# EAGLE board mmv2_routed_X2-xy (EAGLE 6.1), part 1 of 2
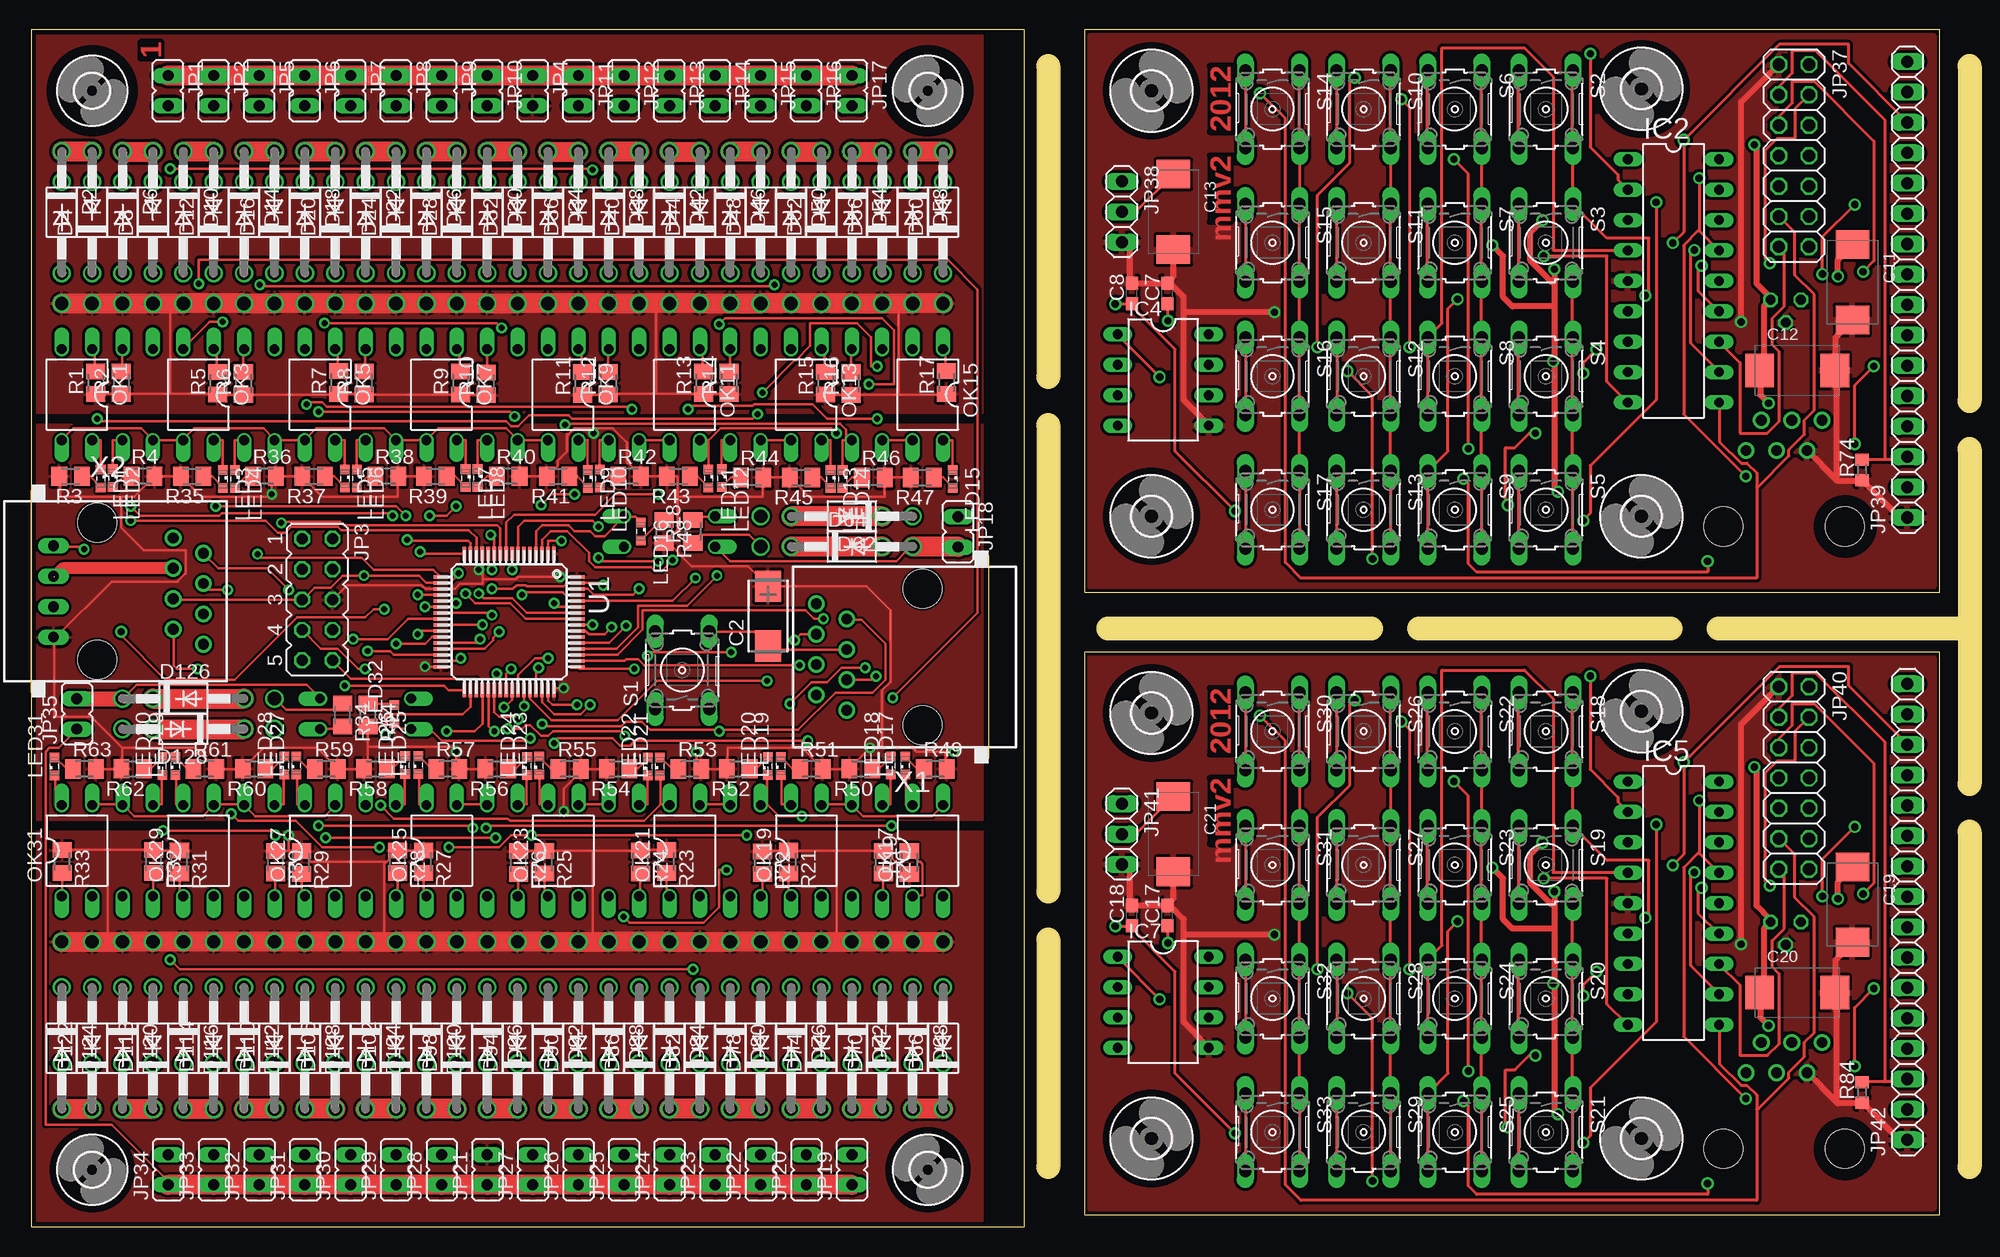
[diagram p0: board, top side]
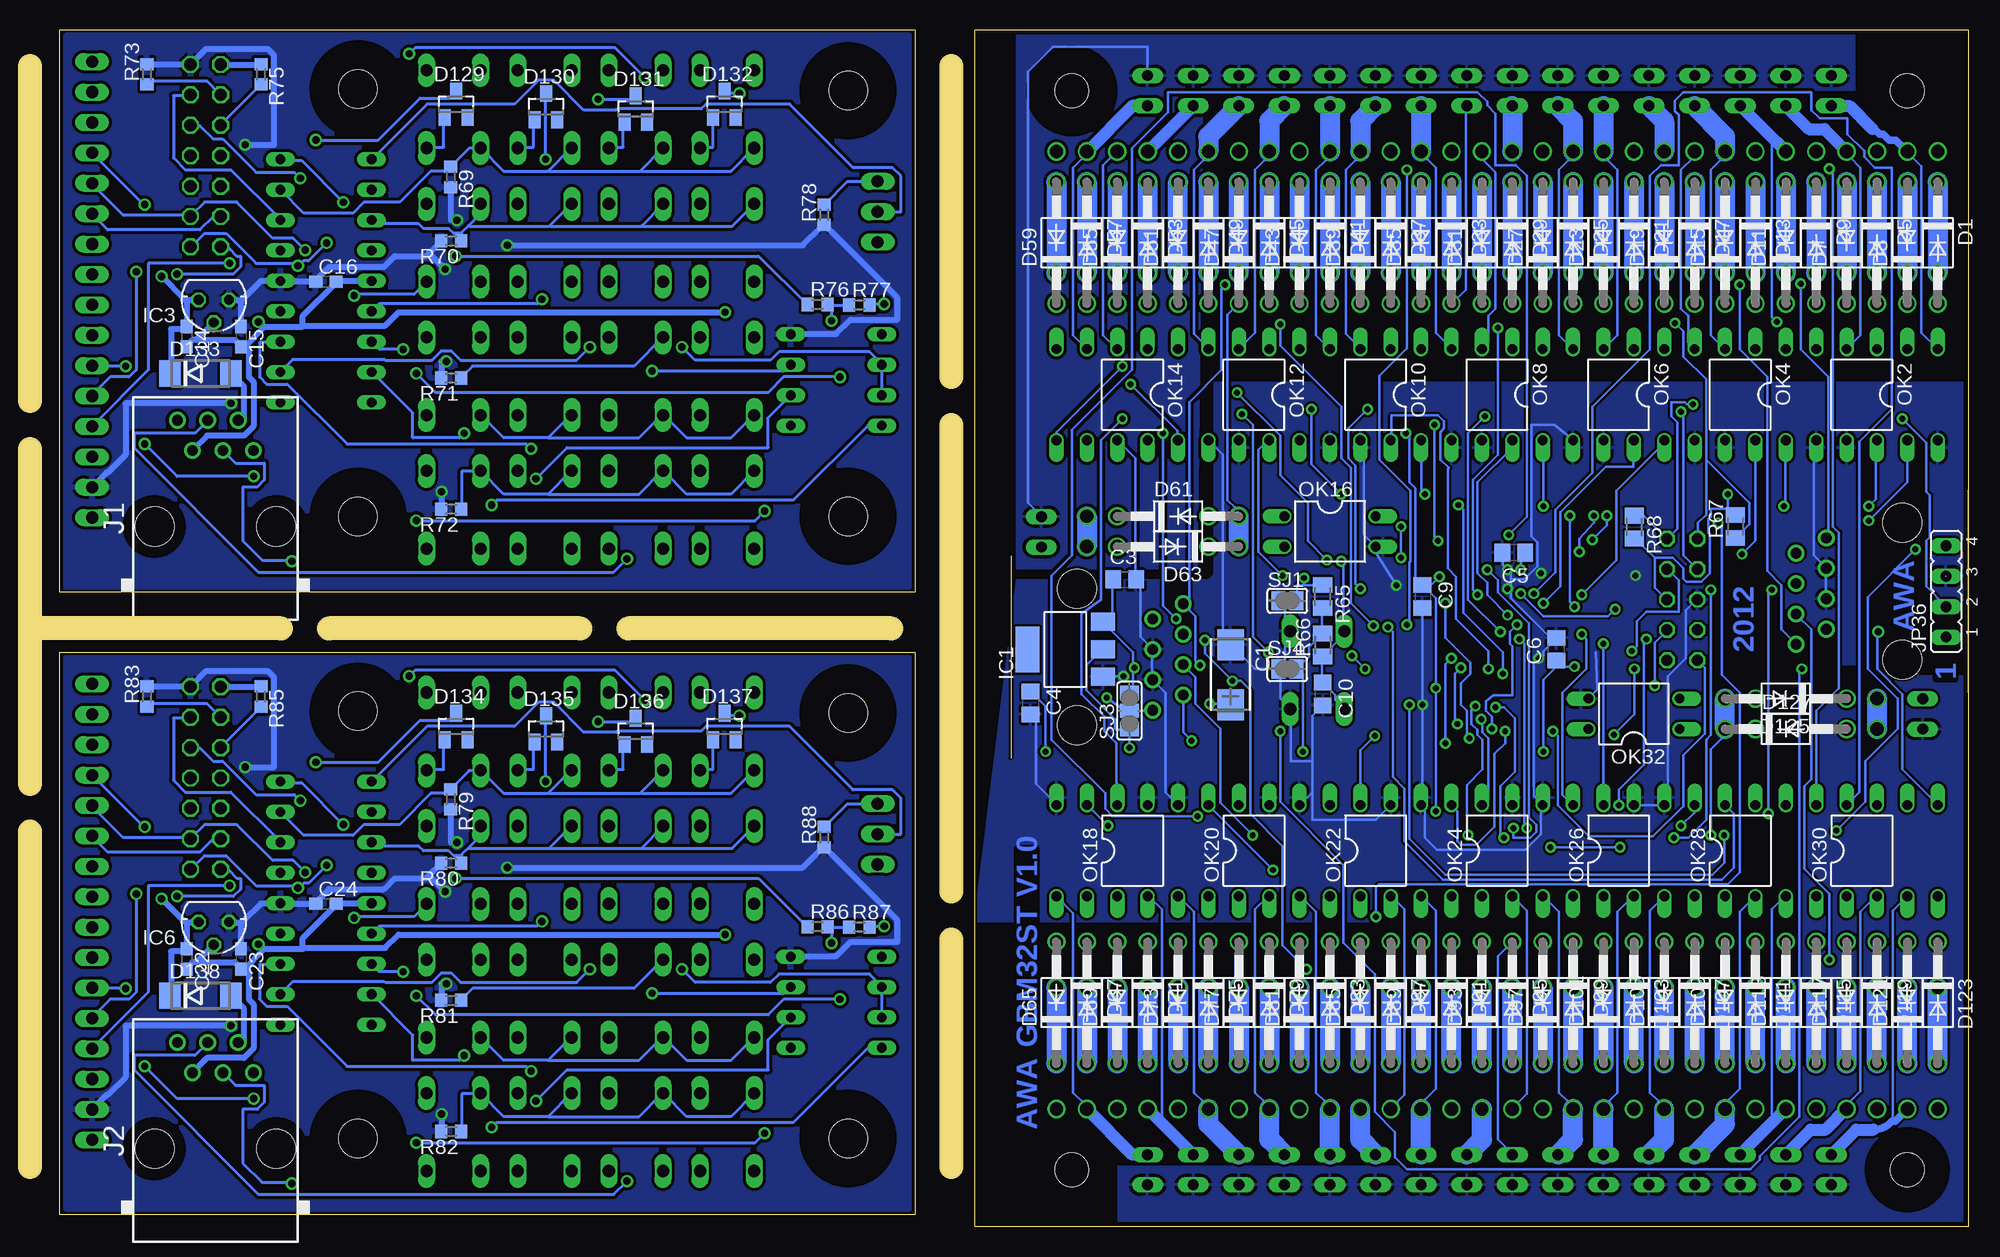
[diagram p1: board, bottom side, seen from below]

Size 162.02 x 100 mm. Coordinates in mm from the lower left corner, seen from the top.
Outline: 90.02,50 112.02,50
Outline: 116.02,50 137.02,50
Outline: 141.02,50 162.02,50
Outline: 162.02,97 162.02,69
Outline: 162.02,65 162.02,37
Outline: 162.02,33 162.02,5
Outline: 85.02,97 85.02,71
Outline: 85.02,67 85.02,28
Outline: 85.02,24 85.02,5
Outline: 0.01,100 0.01,0 83.01,0 83.01,100 0.01,100
Outline: 159.52,100 88.02,100 88.02,53 159.52,53 159.52,100
Outline: 159.52,48 88.02,48 88.02,1 159.52,1 159.52,48
Copper layers (1*16): Top 0.035mm / dielectric 1.5mm / Bottom 0.035mm
Design rules: minimum track width 0.2mm, minimum drill 0.5mm, track to track 0.2mm, track to pad 0.2mm, pad to pad 0.15mm, via to via 0.2mm, smd to smd 0mil, copper to edge 0.2mm, drill to drill 0.2mm, minimum pad ring 0.2mm, minimum via ring 0.2mm, stop-mask expansion 0.1mm, vias tented up to drill 0mil, thermal gap 10mil
Net classes: 1 Power: width 0.508 mm, clearance 0.254 mm

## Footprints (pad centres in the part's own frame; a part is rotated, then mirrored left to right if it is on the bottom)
CT6032 = smd 2.6 x 2.2: + 2.5,0; - -2.5,0
C0805 = smd 1.3 x 1.5: 1 -0.95,0; 2 0.95,0
C0603 = smd 1.1 x 1: 1 -0.85,0; 2 0.85,0
SMC_E = smd 2.4 x 2.8: + -3.15,0; - 3.15,0
DO41-10 = drill 1.118: A 5.08,0; C -5.08,0
SOT23 = smd 1 x 1.4: 1 -0.95,-1.1; 2 0.95,-1.1; 3 0,1.1
DO214AA = smd 1.8 x 2.2: A 2.55,0; C -2.55,0
2,8 = hole 2.8: 0,0
3,2 = hole 3.2: 0,0
SOT223 = smd 1.499 x 2.007: 1 -2.261,-3.15; 2 0.025,-3.15; 3 2.311,-3.15 | smd 3.81 x 2.007: 4 0,3.15
DIL18 = drill 0.813 long: 1 -10.16,-3.81; 2 -7.62,-3.81; 3 -5.08,-3.81; 4 -2.54,-3.81; 5 0,-3.81; 6 2.54,-3.81; 7 5.08,-3.81; 8 7.62,-3.81; 9 10.16,-3.81; 10 10.16,3.81; 11 7.62,3.81; 12 5.08,3.81; 13 2.54,3.81; 14 0,3.81; 15 -2.54,3.81; 16 -5.08,3.81; 17 -7.62,3.81; 18 -10.16,3.81
78LXX = drill 0.813 octagon: GND 0,1.905; IN 1.27,0; OUT -1.27,0
DIL08 = drill 0.813 long: 1 -3.81,-3.81; 2 -1.27,-3.81; 3 1.27,-3.81; 4 3.81,-3.81; 5 3.81,3.81; 6 1.27,3.81; 7 -1.27,3.81; 8 -3.81,3.81
RJ11-NO_SHIELD = drill 0.9 pad 1.4: 1 -3.175,8.89; 2 -1.905,6.35; 3 -0.635,8.89; 4 0.635,6.35; 5 1.905,8.89; 6 3.175,6.35 | hole 3.251: -5.08,0; 5.08,0
JP1 = drill 0.914 long: 1 0,-1.27; 2 0,1.27
JP5Q = drill 0.914 octagon: 1 -5.08,-1.27; 2 -5.08,1.27; 3 -2.54,-1.27; 4 -2.54,1.27; 5 0,-1.27; 6 0,1.27; 7 2.54,-1.27; 8 2.54,1.27; 9 5.08,-1.27; 10 5.08,1.27
JP4 = drill 0.914 long: 1 -3.81,0; 2 -1.27,0; 3 1.27,0; 4 3.81,0
2X07 = drill 1.016 octagon: 1 -7.62,-1.27; 2 -7.62,1.27; 3 -5.08,-1.27; 4 -5.08,1.27; 5 -2.54,-1.27; 6 -2.54,1.27; 7 0,-1.27; 8 0,1.27; 9 2.54,-1.27; 10 2.54,1.27; 11 5.08,-1.27; 12 5.08,1.27; 13 7.62,-1.27; 14 7.62,1.27
1X03 = drill 1.016 long: 1 -2.54,0; 2 0,0; 3 2.54,0
1X16 = drill 1.016 long: 1 -19.05,0; 2 -16.51,0; 3 -13.97,0; 4 -11.43,0; 5 -8.89,0; 6 -6.35,0; 7 -3.81,0; 8 -1.27,0; 9 1.27,0; 10 3.81,0; 11 6.35,0; 12 8.89,0; 13 11.43,0; 14 13.97,0; 15 16.51,0; 16 19.05,0
SML0603 = smd 0.8 x 0.8: A 0.75,0; C -0.75,0
DIL04 = drill 0.813 offset: 1 -1.27,-3.81; 2 1.27,-3.81; 3 1.27,3.81; 4 -1.27,3.81
M0805 = smd 1.3 x 1.6: 1 -0.95,0; 2 0.95,0
R0603 = smd 1 x 1.1: 1 -0.85,0; 2 0.85,0
B3F-10XX = drill 1.016 long: 1 -3.251,2.261; 2 3.251,2.261; 3 -3.251,-2.261; 4 3.251,-2.261
SJ = smd 1.168 x 1.6: 1 -0.762,0; 2 0.762,0
SJ_2 = smd 1.168 x 1.6: 1 -1.524,0; 2 0,0; 3 1.524,0
TQFP64 = smd 1.2 x 0.3: 1 -5.7,3.75; 2 -5.7,3.25; 3 -5.7,2.75; 4 -5.7,2.25; 5 -5.7,1.75; 6 -5.7,1.25; 7 -5.7,0.75; 8 -5.7,0.25; 9 -5.7,-0.25; 10 -5.7,-0.75; 11 -5.7,-1.25; 12 -5.7,-1.75; 13 -5.7,-2.25; 14 -5.7,-2.75; 15 -5.7,-3.25; 16 -5.7,-3.75; 33 5.7,-3.75; 34 5.7,-3.25; 35 5.7,-2.75; 36 5.7,-2.25; 37 5.7,-1.75; 38 5.7,-1.25; 39 5.7,-0.75; 40 5.7,-0.25; 41 5.7,0.25; 42 5.7,0.75; 43 5.7,1.25; 44 5.7,1.75; 45 5.7,2.25; 46 5.7,2.75; 47 5.7,3.25; 48 5.7,3.75 | smd 0.3 x 1.2: 17 -3.75,-5.7; 18 -3.25,-5.7; 19 -2.75,-5.7; 20 -2.25,-5.7; 21 -1.75,-5.7; 22 -1.25,-5.7; 23 -0.75,-5.7; 24 -0.25,-5.7; 25 0.25,-5.7; 26 0.75,-5.7; 27 1.25,-5.7; 28 1.75,-5.7; 29 2.25,-5.7; 30 2.75,-5.7; 31 3.25,-5.7; 32 3.75,-5.7; 49 3.75,5.7; 50 3.25,5.7; 51 2.75,5.7; 52 2.25,5.7; 53 1.75,5.7; 54 1.25,5.7; 55 0.75,5.7; 56 0.25,5.7; 57 -0.25,5.7; 58 -0.75,5.7; 59 -1.25,5.7; 60 -1.75,5.7; 61 -2.25,5.7; 62 -2.75,5.7; 63 -3.25,5.7; 64 -3.75,5.7
RJ45-NO-SHIELD = drill 0.9 pad 1.4: 1 -4.445,6.35; 2 -3.175,8.89; 3 -1.905,6.35; 4 -0.635,8.89; 5 0.635,6.35; 6 1.905,8.89; 7 3.175,6.35; 8 4.445,8.89 | hole 3.251: -5.715,0; 5.715,0

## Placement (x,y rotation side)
C1  [CT6032]  61.66,46.12 270 bottom
C2  [CT6032]  61.58,51.02 90 top
C3  [C0805]  70.5,54.08 0 bottom
C4  [C0805]  78.37,43.75 270 bottom
C5  [C0805]  37.99,56.32 180 bottom
C6  [C0805]  34.42,48.24 90 bottom
C7  100nF  [C0603]  94.96,77.98 90 top
C8  100nF  [C0603]  92,77.98 90 top
C9  [C0805]  45.61,52.65 270 bottom
C10  [C0805]  53.96,44.5 270 bottom
C11  100µF  [SMC_E]  152.23,78.91 270 top
C12  100µF  [SMC_E]  147.61,71.55 0 top
C13  10µF  [SMC_E]  95.47,84.8 270 top
C14  100nF  [C0603]  148.92,74.37 270 bottom
C15  100nF  [C0603]  144.38,74.37 270 bottom
C16  100nF  [C0603]  137.27,78.97 0 bottom
C17  100nF  [C0603]  94.96,25.98 90 top
C18  100nF  [C0603]  92,25.98 90 top
C19  100µF  [SMC_E]  152.23,26.91 270 top
C20  100µF  [SMC_E]  147.61,19.55 0 top
C21  10µF  [SMC_E]  95.47,32.8 270 top
C22  100nF  [C0603]  148.92,22.37 270 bottom
C23  100nF  [C0603]  144.38,22.37 270 bottom
C24  100nF  [C0603]  137.27,26.97 0 bottom
D1  1N4004  [DO41-10]  2.55,82.22 270 bottom
D2  1N4004  [DO41-10]  2.55,84.76 270 top
D3  1N4004  [DO41-10]  5.09,82.22 90 bottom
D4  1N4004  [DO41-10]  5.09,84.76 90 top
D5  1N4004  [DO41-10]  7.63,82.22 270 bottom
D6  1N4004  [DO41-10]  7.63,84.76 270 top
D7  1N4004  [DO41-10]  10.17,82.22 90 bottom
D8  1N4004  [DO41-10]  10.17,84.76 90 top
D9  1N4004  [DO41-10]  12.71,82.22 270 bottom
D10  1N4004  [DO41-10]  12.71,84.76 270 top
D11  1N4004  [DO41-10]  15.25,82.22 90 bottom
D12  1N4004  [DO41-10]  15.25,84.76 90 top
D13  1N4004  [DO41-10]  17.79,82.22 270 bottom
D14  1N4004  [DO41-10]  17.79,84.76 270 top
D15  1N4004  [DO41-10]  20.33,82.22 90 bottom
D16  1N4004  [DO41-10]  20.33,84.76 90 top
D17  1N4004  [DO41-10]  22.87,82.22 270 bottom
D18  1N4004  [DO41-10]  22.87,84.76 270 top
D19  1N4004  [DO41-10]  25.41,82.22 90 bottom
D20  1N4004  [DO41-10]  25.41,84.76 90 top
D21  1N4004  [DO41-10]  27.95,82.22 270 bottom
D22  1N4004  [DO41-10]  27.95,84.76 270 top
D23  1N4004  [DO41-10]  30.49,82.22 90 bottom
D24  1N4004  [DO41-10]  30.49,84.76 90 top
D25  1N4004  [DO41-10]  33.03,82.22 270 bottom
D26  1N4004  [DO41-10]  33.03,84.76 270 top
D27  1N4004  [DO41-10]  35.57,82.22 90 bottom
D28  1N4004  [DO41-10]  35.57,84.76 90 top
D29  1N4004  [DO41-10]  38.11,82.22 270 bottom
D30  1N4004  [DO41-10]  38.11,84.76 270 top
D31  1N4004  [DO41-10]  40.65,82.22 90 bottom
D32  1N4004  [DO41-10]  40.65,84.76 90 top
D33  1N4004  [DO41-10]  43.19,82.22 270 bottom
D34  1N4004  [DO41-10]  43.19,84.76 270 top
D35  1N4004  [DO41-10]  45.73,82.22 90 bottom
D36  1N4004  [DO41-10]  45.73,84.76 90 top
D37  1N4004  [DO41-10]  48.27,82.22 270 bottom
D38  1N4004  [DO41-10]  48.27,84.76 270 top
D39  1N4004  [DO41-10]  50.81,82.22 90 bottom
D40  1N4004  [DO41-10]  50.81,84.76 90 top
D41  1N4004  [DO41-10]  53.35,82.22 270 bottom
D42  1N4004  [DO41-10]  53.35,84.76 270 top
D43  1N4004  [DO41-10]  55.89,82.22 90 bottom
D44  1N4004  [DO41-10]  55.89,84.76 90 top
D45  1N4004  [DO41-10]  58.43,82.22 270 bottom
D46  1N4004  [DO41-10]  58.43,84.76 270 top
D47  1N4004  [DO41-10]  60.97,82.22 90 bottom
D48  1N4004  [DO41-10]  60.97,84.76 90 top
D49  1N4004  [DO41-10]  63.51,82.22 270 bottom
D50  1N4004  [DO41-10]  63.51,84.76 270 top
D51  1N4004  [DO41-10]  66.05,82.22 90 bottom
D52  1N4004  [DO41-10]  66.05,84.76 90 top
D53  1N4004  [DO41-10]  68.59,82.22 270 bottom
D54  1N4004  [DO41-10]  68.59,84.76 270 top
D55  1N4004  [DO41-10]  71.13,82.22 90 bottom
D56  1N4004  [DO41-10]  71.13,84.76 90 top
D57  1N4004  [DO41-10]  73.67,82.22 270 bottom
D58  1N4004  [DO41-10]  73.67,84.76 270 top
D59  1N4004  [DO41-10]  76.21,82.22 90 bottom
D60  1N4004  [DO41-10]  76.21,84.76 90 top
D61  1N4004  [DO41-10]  66.05,59.36 0 bottom
D62  1N4004  [DO41-10]  68.59,59.36 180 top
D63  1N4004  [DO41-10]  66.05,56.82 180 bottom
D64  1N4004  [DO41-10]  68.59,56.82 0 top
D65  1N4004  [DO41-10]  76.21,18.72 90 bottom
D66  1N4004  [DO41-10]  76.21,14.91 90 top
D67  1N4004  [DO41-10]  73.67,18.72 270 bottom
D68  1N4004  [DO41-10]  73.67,14.91 270 top
D69  1N4004  [DO41-10]  71.13,18.72 90 bottom
D70  1N4004  [DO41-10]  71.13,14.91 90 top
D71  1N4004  [DO41-10]  68.59,18.72 270 bottom
D72  1N4004  [DO41-10]  68.59,14.91 270 top
D73  1N4004  [DO41-10]  66.05,18.72 90 bottom
D74  1N4004  [DO41-10]  66.05,14.91 90 top
D75  1N4004  [DO41-10]  63.51,18.72 270 bottom
D76  1N4004  [DO41-10]  63.51,14.91 270 top
D77  1N4004  [DO41-10]  60.97,18.72 90 bottom
D78  1N4004  [DO41-10]  60.97,14.91 90 top
D79  1N4004  [DO41-10]  58.43,18.72 270 bottom
D80  1N4004  [DO41-10]  58.43,14.91 270 top
D81  1N4004  [DO41-10]  55.89,18.72 90 bottom
D82  1N4004  [DO41-10]  55.89,14.91 90 top
D83  1N4004  [DO41-10]  53.35,18.72 270 bottom
D84  1N4004  [DO41-10]  53.35,14.91 270 top
D85  1N4004  [DO41-10]  50.81,18.72 90 bottom
D86  1N4004  [DO41-10]  50.81,14.91 90 top
D87  1N4004  [DO41-10]  48.27,18.72 270 bottom
D88  1N4004  [DO41-10]  48.27,14.91 270 top
D89  1N4004  [DO41-10]  45.73,18.72 90 bottom
D90  1N4004  [DO41-10]  45.73,14.91 90 top
D91  1N4004  [DO41-10]  43.19,18.72 270 bottom
D92  1N4004  [DO41-10]  43.19,14.91 270 top
D93  1N4004  [DO41-10]  40.65,18.72 90 bottom
D94  1N4004  [DO41-10]  40.65,14.91 90 top
D95  1N4004  [DO41-10]  38.11,18.72 270 bottom
D96  1N4004  [DO41-10]  38.11,14.91 270 top
D97  1N4004  [DO41-10]  35.57,18.72 90 bottom
D98  1N4004  [DO41-10]  35.57,14.91 90 top
D99  1N4004  [DO41-10]  33.03,18.72 270 bottom
D100  1N4004  [DO41-10]  33.03,14.91 270 top
D101  1N4004  [DO41-10]  30.49,18.72 90 bottom
D102  1N4004  [DO41-10]  30.49,14.91 90 top
D103  1N4004  [DO41-10]  27.95,18.72 270 bottom
D104  1N4004  [DO41-10]  27.95,14.91 270 top
D105  1N4004  [DO41-10]  25.41,18.72 90 bottom
D106  1N4004  [DO41-10]  25.41,14.91 90 top
D107  1N4004  [DO41-10]  22.87,18.72 270 bottom
D108  1N4004  [DO41-10]  22.87,14.91 270 top
D109  1N4004  [DO41-10]  20.33,18.72 90 bottom
D110  1N4004  [DO41-10]  20.33,14.91 90 top
D111  1N4004  [DO41-10]  17.79,18.72 270 bottom
D112  1N4004  [DO41-10]  17.79,14.91 270 top
D113  1N4004  [DO41-10]  15.25,18.72 90 bottom
D114  1N4004  [DO41-10]  15.25,14.91 90 top
D115  1N4004  [DO41-10]  12.71,18.72 270 bottom
D116  1N4004  [DO41-10]  12.71,14.91 270 top
D117  1N4004  [DO41-10]  10.17,18.72 90 bottom
D118  1N4004  [DO41-10]  10.17,14.91 90 top
D119  1N4004  [DO41-10]  7.63,18.72 270 bottom
D120  1N4004  [DO41-10]  7.63,14.91 270 top
D121  1N4004  [DO41-10]  5.09,18.72 90 bottom
D122  1N4004  [DO41-10]  5.09,14.91 90 top
D123  1N4004  [DO41-10]  2.55,18.72 270 bottom
D124  1N4004  [DO41-10]  2.55,14.91 270 top
D125  1N4004  [DO41-10]  15.25,44.12 180 bottom
D126  1N4004  [DO41-10]  12.71,44.12 0 top
D127  1N4004  [DO41-10]  15.25,41.58 0 bottom
D128  1N4004  [DO41-10]  12.71,41.58 180 top
D129  BAV199  [SOT23]  126.4,93.79 0 bottom
D130  BAV199  [SOT23]  118.89,93.59 0 bottom
D131  BAV199  [SOT23]  111.38,93.39 0 bottom
D132  BAV199  [SOT23]  103.97,93.79 0 bottom
D133  [DO214AA]  147.76,71.29 0 bottom
D134  BAV199  [SOT23]  126.4,41.79 0 bottom
D135  BAV199  [SOT23]  118.89,41.59 0 bottom
D136  BAV199  [SOT23]  111.38,41.39 0 bottom
D137  BAV199  [SOT23]  103.97,41.79 0 bottom
D138  [DO214AA]  147.76,19.29 0 bottom
H1  MOUNT-HOLE2.8  [2,8]  5.09,94.92 270 top
H2  MOUNT-HOLE2.8  [2,8]  74.94,94.92 270 top
H3  MOUNT-HOLE2.8  [2,8]  5.09,4.75 270 top
H4  MOUNT-HOLE2.8  [2,8]  74.94,4.75 270 top
H5  MOUNT-HOLE3.2  [3,2]  134.59,59.36 180 top
H6  MOUNT-HOLE3.2  [3,2]  93.63,59.36 180 top
H7  MOUNT-HOLE3.2  [3,2]  134.59,95.07 180 top
H8  MOUNT-HOLE3.2  [3,2]  93.63,94.92 180 top
H9  MOUNT-HOLE3.2  [3,2]  134.59,7.36 180 top
H10  MOUNT-HOLE3.2  [3,2]  93.63,7.36 180 top
H11  MOUNT-HOLE3.2  [3,2]  134.59,43.07 180 top
H12  MOUNT-HOLE3.2  [3,2]  93.63,42.92 180 top
IC1  REG1117  [SOT223]  75.48,48.22 90 bottom
IC2  PIC16F628P  [DIL18]  137.27,79.03 270 top
IC3  [78LXX]  146.65,77.45 180 bottom
IC4  MAX481CPA  [DIL08]  94.62,70.75 270 top
IC5  PIC16F628P  [DIL18]  137.27,27.03 270 top
IC6  [78LXX]  146.65,25.45 180 bottom
IC7  MAX481CPA  [DIL08]  94.62,18.75 270 top
J1  RJ11-6L-B  [RJ11-NO_SHIELD]  146.52,58.5 0 bottom
J2  RJ11-6L-B  [RJ11-NO_SHIELD]  146.52,6.5 0 bottom
JP1  [JP1]  11.44,94.92 180 top
JP2  [JP1]  15.25,94.92 180 top
JP3  [JP5Q]  23.91,52.4 270 top
JP4  [JP1]  41.92,94.92 180 top
JP5  [JP1]  19.06,94.92 180 top
JP6  [JP1]  22.87,94.92 180 top
JP7  [JP1]  26.68,94.92 180 top
JP8  [JP1]  30.49,94.92 180 top
JP9  [JP1]  34.3,94.92 180 top
JP10  [JP1]  38.11,94.92 180 top
JP11  [JP1]  45.73,94.92 180 top
JP12  [JP1]  49.54,94.92 180 top
JP13  [JP1]  53.35,94.92 180 top
JP14  [JP1]  57.16,94.92 180 top
JP15  [JP1]  60.97,94.92 180 top
JP16  [JP1]  64.78,94.92 180 top
JP17  [JP1]  68.59,94.92 180 top
JP18  [JP1]  77.48,58.06 180 top
JP19  [JP1]  68.59,4.75 0 top
JP20  [JP1]  64.78,4.75 0 top
JP21  [JP1]  38.11,4.75 0 top
JP22  [JP1]  60.97,4.75 0 top
JP23  [JP1]  57.16,4.75 0 top
JP24  [JP1]  53.35,4.75 0 top
JP25  [JP1]  49.54,4.75 0 top
JP26  [JP1]  45.73,4.75 0 top
JP27  [JP1]  41.92,4.75 0 top
JP28  [JP1]  34.3,4.75 0 top
JP29  [JP1]  30.49,4.75 0 top
JP30  [JP1]  26.68,4.75 0 top
JP31  [JP1]  22.87,4.75 0 top
JP32  [JP1]  19.06,4.75 0 top
JP33  [JP1]  15.25,4.75 0 top
JP34  [JP1]  11.44,4.75 0 top
JP35  [JP1]  3.82,42.85 0 top
JP36  [JP4]  1.86,53.08 90 bottom
JP37  [2X07]  147.33,89.49 270 top
JP38  [1X03]  91.16,84.8 270 top
JP39  [1X16]  156.82,78.3 90 top
JP40  [2X07]  147.33,37.49 270 top
JP41  [1X03]  91.16,32.8 270 top
JP42  [1X16]  156.82,26.3 90 top
LED1  [SML0603]  5.81,62.52 270 top
LED2  [SML0603]  6.81,62.54 270 top
LED3  [SML0603]  16.01,62.46 270 top
LED4  [SML0603]  17.01,62.48 270 top
LED5  [SML0603]  26.21,62.5 270 top
LED6  [SML0603]  27.21,62.52 270 top
LED7  [SML0603]  36.31,62.54 270 top
LED8  [SML0603]  37.31,62.56 270 top
LED9  [SML0603]  46.51,62.48 270 top
LED10  [SML0603]  47.51,62.5 270 top
LED11  [SML0603]  56.61,62.52 270 top
LED12  [SML0603]  57.71,62.54 270 top
LED13  [SML0603]  66.81,62.46 270 top
LED14  [SML0603]  67.81,62.48 270 top
LED15  [SML0603]  77.01,62.47 270 top
LED16  [SML0603]  50.96,58.09 270 top
LED17  [SML0603]  73.05,38.54 90 top
LED18  [SML0603]  71.85,38.52 90 top
LED19  [SML0603]  62.65,38.5 90 top
LED20  [SML0603]  61.55,38.48 90 top
LED21  [SML0603]  52.55,38.46 90 top
LED22  [SML0603]  51.55,38.44 90 top
LED23  [SML0603]  42.45,38.52 90 top
LED24  [SML0603]  41.45,38.5 90 top
LED25  [SML0603]  32.35,38.58 90 top
LED26  [SML0603]  31.25,38.56 90 top
LED27  [SML0603]  22.15,38.54 90 top
LED28  [SML0603]  21.15,38.52 90 top
LED29  [SML0603]  12.05,38.5 90 top
LED30  [SML0603]  10.95,38.48 90 top
LED31  [SML0603]  1.95,38.46 90 top
LED32  [SML0603]  30.37,42.85 90 top
OK1  PC817  [DIL04]  3.82,69.52 180 top
OK2  PC817  [DIL04]  8.9,69.52 180 bottom
OK3  PC817  [DIL04]  13.98,69.52 180 top
OK4  PC817  [DIL04]  19.06,69.52 180 bottom
OK5  PC817  [DIL04]  24.14,69.52 180 top
OK6  PC817  [DIL04]  29.22,69.52 180 bottom
OK7  PC817  [DIL04]  34.3,69.52 180 top
OK8  PC817  [DIL04]  39.38,69.52 180 bottom
OK9  PC817  [DIL04]  44.46,69.52 180 top
OK10  PC817  [DIL04]  49.54,69.52 180 bottom
OK11  PC817  [DIL04]  54.62,69.52 180 top
OK12  PC817  [DIL04]  59.7,69.52 180 bottom
OK13  PC817  [DIL04]  64.78,69.52 180 top
OK14  PC817  [DIL04]  69.86,69.52 180 bottom
OK15  PC817  [DIL04]  74.94,69.52 180 top
OK16  PC817  [DIL04]  53.35,58.09 270 bottom
OK17  PC817  [DIL04]  74.94,31.42 0 top
OK18  PC817  [DIL04]  69.86,31.42 0 bottom
OK19  PC817  [DIL04]  64.78,31.42 0 top
OK20  PC817  [DIL04]  59.7,31.42 0 bottom
OK21  PC817  [DIL04]  54.62,31.42 0 top
OK22  PC817  [DIL04]  49.54,31.42 0 bottom
OK23  PC817  [DIL04]  44.46,31.42 0 top
OK24  PC817  [DIL04]  39.38,31.42 0 bottom
OK25  PC817  [DIL04]  34.3,31.42 0 top
OK26  PC817  [DIL04]  29.22,31.42 0 bottom
OK27  PC817  [DIL04]  24.14,31.42 0 top
OK28  PC817  [DIL04]  19.06,31.42 0 bottom
OK29  PC817  [DIL04]  13.98,31.42 0 top
OK30  PC817  [DIL04]  8.9,31.42 0 bottom
OK31  PC817  [DIL04]  3.82,31.42 0 top
OK32  PC817  [DIL04]  27.95,42.85 90 bottom
R1  680R  [M0805]  5.39,70.51 90 top
R2  680R  [M0805]  7.53,70.51 90 top
R3  [M0805]  3.29,62.7 180 top
R4  [M0805]  9.35,62.7 0 top
R5  680R  [M0805]  15.59,70.47 90 top
R6  680R  [M0805]  17.73,70.45 90 top
R7  680R  [M0805]  25.69,70.53 90 top
R8  680R  [M0805]  27.83,70.49 90 top
R9  680R  [M0805]  35.89,70.49 90 top
R10  680R  [M0805]  38.03,70.43 90 top
R11  680R  [M0805]  46.09,70.45 90 top
R12  680R  [M0805]  48.23,70.47 90 top
R13  680R  [M0805]  56.19,70.51 90 top
R14  680R  [M0805]  58.33,70.51 90 top
R15  680R  [M0805]  66.39,70.47 90 top
R16  680R  [M0805]  68.53,70.45 90 top
R17  680R  [M0805]  76.49,70.53 90 top
R18  680R  [M0805]  55.3,58.09 90 top
R19  680R  [M0805]  73.39,30.43 90 top
R20  680R  [M0805]  71.23,30.45 270 top
R21  680R  [M0805]  63.29,30.47 270 top
R22  680R  [M0805]  61.13,30.41 270 top
R23  680R  [M0805]  53.09,30.51 270 top
R24  680R  [M0805]  50.93,30.47 270 top
R25  680R  [M0805]  42.89,30.45 270 top
R26  680R  [M0805]  40.73,30.43 270 top
R27  680R  [M0805]  32.79,30.49 270 top
R28  680R  [M0805]  30.63,30.49 270 top
R29  680R  [M0805]  22.59,30.43 270 top
R30  680R  [M0805]  20.43,30.45 270 top
R31  680R  [M0805]  12.39,30.47 270 top
R32  680R  [M0805]  10.23,30.51 270 top
R33  680R  [M0805]  2.59,30.51 270 top
R34  680R  [M0805]  26.02,42.75 270 top
R35  [M0805]  13.45,62.7 180 top
R36  [M0805]  19.49,62.7 0 top
R37  [M0805]  23.61,62.7 180 top
R38  [M0805]  29.73,62.7 0 top
R39  [M0805]  33.77,62.7 180 top
R40  [M0805]  39.87,62.7 0 top
R41  [M0805]  44.03,62.7 180 top
R42  [M0805]  50.01,62.7 0 top
R43  [M0805]  54.09,62.7 180 top
R44  [M0805]  60.25,62.6 0 top
R45  [M0805]  64.35,62.6 180 top
R46  [M0805]  70.39,62.6 0 top
R47  [M0805]  74.48,62.6 180 top
R48  [M0805]  52.91,58.09 270 top
R49  [M0805]  75.57,38.24 0 top
R50  [M0805]  69.33,38.26 180 top
R51  [M0805]  65.21,38.24 0 top
R52  [M0805]  59.09,38.26 180 top
R53  [M0805]  55.05,38.24 0 top
R54  [M0805]  49.05,38.26 180 top
R55  [M0805]  44.99,38.24 0 top
R56  [M0805]  38.91,38.26 180 top
R57  [M0805]  34.83,38.24 0 top
R58  [M0805]  28.77,38.26 180 top
R59  [M0805]  24.67,38.24 0 top
R60  [M0805]  18.63,38.26 180 top
R61  [M0805]  14.51,38.24 0 top
R62  [M0805]  8.49,38.26 180 top
R63  [M0805]  4.45,38.24 0 top
R64  [M0805]  28.15,42.75 270 top
R65  10k  [M0805]  53.96,52.65 270 bottom
R66  10k  [M0805]  53.96,48.6 90 bottom
R67  10k  [M0805]  19.46,58.5 90 bottom
R68  10k  [M0805]  27.91,58.45 270 bottom
R69  10k  [R0603]  126.85,87.71 270 bottom
R70  10k  [R0603]  126.81,82.37 180 bottom
R71  10k  [R0603]  126.81,70.91 180 bottom
R72  10k  [R0603]  126.81,59.95 180 bottom
R73  10k  [R0603]  152.24,96.3 90 bottom
R74  330R  [R0603]  153.03,63.22 90 top
R75  0R  [R0603]  142.7,96.3 270 bottom
R76  2k7  [R0603]  96.19,77.06 0 bottom
R77  2k7  [R0603]  92.69,77.02 0 bottom
R78  5k6  [R0603]  95.63,84.55 90 bottom
R79  10k  [R0603]  126.85,35.71 270 bottom
R80  10k  [R0603]  126.81,30.37 180 bottom
R81  10k  [R0603]  126.81,18.91 180 bottom
R82  10k  [R0603]  126.81,7.95 180 bottom
R83  10k  [R0603]  152.24,44.3 90 bottom
R84  330R  [R0603]  153.03,11.22 90 top
R85  0R  [R0603]  142.7,44.3 270 bottom
R86  2k7  [R0603]  96.19,25.06 0 bottom
R87  2k7  [R0603]  92.69,25.02 0 bottom
R88  5k6  [R0603]  95.63,32.55 90 bottom
S1  [B3F-10XX]  54.41,46.5 90 top
S2  [B3F-10XX]  126.61,93.38 270 top
S3  [B3F-10XX]  126.61,82.22 270 top
S4  [B3F-10XX]  126.61,71.06 270 top
S5  [B3F-10XX]  126.61,59.9 270 top
S6  [B3F-10XX]  118.99,93.38 270 top
S7  [B3F-10XX]  118.99,82.22 270 top
S8  [B3F-10XX]  118.99,71.06 270 top
S9  [B3F-10XX]  118.99,59.9 270 top
S10  [B3F-10XX]  111.37,93.38 270 top
S11  [B3F-10XX]  111.37,82.22 270 top
S12  [B3F-10XX]  111.37,71.06 270 top
S13  [B3F-10XX]  111.37,59.9 270 top
S14  [B3F-10XX]  103.75,93.38 270 top
S15  [B3F-10XX]  103.75,82.22 270 top
S16  [B3F-10XX]  103.75,71.06 270 top
S17  [B3F-10XX]  103.75,59.9 270 top
S18  [B3F-10XX]  126.61,41.38 270 top
S19  [B3F-10XX]  126.61,30.22 270 top
S20  [B3F-10XX]  126.61,19.06 270 top
S21  [B3F-10XX]  126.61,7.9 270 top
S22  [B3F-10XX]  118.99,41.38 270 top
S23  [B3F-10XX]  118.99,30.22 270 top
S24  [B3F-10XX]  118.99,19.06 270 top
S25  [B3F-10XX]  118.99,7.9 270 top
S26  [B3F-10XX]  111.37,41.38 270 top
S27  [B3F-10XX]  111.37,30.22 270 top
S28  [B3F-10XX]  111.37,19.06 270 top
S29  [B3F-10XX]  111.37,7.9 270 top
S30  [B3F-10XX]  103.75,41.38 270 top
S31  [B3F-10XX]  103.75,30.22 270 top
S32  [B3F-10XX]  103.75,19.06 270 top
S33  [B3F-10XX]  103.75,7.9 270 top
SJ1  [SJ]  56.91,52.3 0 bottom
SJ3  [SJ_2]  70.11,43.1 90 bottom
SJ4  [SJ]  56.91,46.6 0 bottom
U1  STM32F10XRXT6  [TQFP64]  39.94,50.53 270 top
X1  RJ45-6L-B  [RJ45-NO-SHIELD]  74.51,47.6 90 top
X2  RJ45-6L-B  [RJ45-NO-SHIELD]  5.51,53.1 270 top

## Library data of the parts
C1 C2 R1-R68 = resistor
C3-C24 R69-R88 = rcl
D1-D138 = diode
H1-H12 = holes
IC1 = burr-brown; MPN: REG1117; OC_FARNELL: 1097566; OC_NEWARK: 14P6981
IC2 IC5 = microchip; MF: MICROCHIP; MPN: PIC16F628-20/P; OC_FARNELL: 9760423; OC_NEWARK: 23C4982
IC3 IC6 = v-reg
IC4 IC7 = maxim; MPN: MAX481CPA+; OC_FARNELL: unknown; OC_NEWARK: 99K3445
J1 J2 = con-tycoelectronics_local; MF: TYCO ELECTRONICS; MPN: RJ11-6L-B; OC_FARNELL: unknown; OC_NEWARK: 52K3613
JP1-JP36 SJ1 SJ3 SJ4 = jumper
JP37-JP42 = pinhead
LED1-LED32 = led
OK1-OK32 = optocoupler; MPN: PC817X4J000F; OC_FARNELL: 9707727; OC_NEWARK: 97K7059
S1-S33 = switch-omron; MPN: B3F-1000; OC_FARNELL: 176432; OC_NEWARK: 36M3542
U1 = stm32
X1 X2 = con-tycoelectronics; MPN: RJ45-6L-B; OC_FARNELL: unknown; OC_NEWARK: 16R6090

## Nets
COL1: IC2.17 R69.1 S2.3 S2.4 S6.3 S6.4 S10.3 S10.4 S14.3 S14.4
COL2: IC2.3 R70.1 S3.3 S3.4 S7.3 S7.4 S11.3 S11.4 S15.3 S15.4
COL3: IC2.4 R71.1 S4.3 S4.4 S8.3 S8.4 S12.3 S12.4 S16.3 S16.4
COL4: IC2.6 R72.1 S5.3 S5.4 S9.3 S9.4 S13.3 S13.4 S17.3 S17.4
COL5: IC5.17 R79.1 S18.3 S18.4 S22.3 S22.4 S26.3 S26.4 S30.3 S30.4
COL6: IC5.3 R80.1 S19.3 S19.4 S23.3 S23.4 S27.3 S27.4 S31.3 S31.4
COL7: IC5.4 R81.1 S20.3 S20.4 S24.3 S24.4 S28.3 S28.4 S32.3 S32.4
COL8: IC5.6 R82.1 S21.3 S21.4 S25.3 S25.4 S29.3 S29.4 S33.3 S33.4
DB1: D137.3 IC5.10 JP40.11 JP42.11
DB2: D135.3 IC5.12 JP40.13 JP42.13
DB3: D136.3 IC5.11 JP40.12 JP42.12
DB4: D132.3 IC2.10 JP37.11 JP39.11
DB5: D131.3 IC2.11 JP37.12 JP39.12
DB6: D130.3 IC2.12 JP37.13 JP39.13
DB7: D129.3 IC2.13 JP37.14 JP39.14
DB8: D134.3 IC5.13 JP40.14 JP42.14
DIR: IC2.2 IC4.2 IC4.3
DIR1: IC5.2 IC7.2 IC7.3
E: IC2.15 JP37.6 JP39.6
E1: IC5.15 JP40.6 JP42.6
GBM0: LED1.C OK1.4 U1.14
GBM1: LED2.C OK2.4 U1.15
GBM2: LED3.C OK3.4 U1.16
GBM3: LED4.C OK4.4 U1.17
GBM4: LED5.C OK5.4 U1.20
GBM5: LED6.C OK6.4 U1.21
GBM6: LED7.C OK7.4 U1.22
GBM7: LED8.C OK8.4 U1.23
GBM8: LED9.C OK9.4 U1.39
GBM9: LED10.C OK10.4 U1.40
GBM10: LED11.C OK11.4 U1.51
GBM11: LED12.C OK12.4 U1.52
GBM12: LED13.C OK13.4 U1.53
GBM13: LED14.C OK14.4 U1.2
GBM14: LED15.C OK15.4 U1.3
GBM15: LED16.C OK16.4 U1.4
GBM16: LED17.C OK17.4 U1.8
GBM17: LED18.C OK18.4 U1.9
GBM18: LED19.C OK19.4 U1.10
GBM19: LED20.C OK20.4 U1.11
GBM20: LED21.C OK21.4 U1.24
GBM21: LED22.C OK22.4 U1.25
GBM22: LED23.C OK23.4 U1.37
GBM23: LED24.C OK24.4 U1.38
GBM24: LED25.C OK25.4 U1.26
GBM25: LED26.C OK26.4 U1.27
GBM26: LED27.C OK27.4 U1.28
GBM27: LED28.C OK28.4 U1.55
GBM28: LED29.C OK29.4 U1.56
GBM29: LED30.C OK30.4 U1.57
GBM30: LED31.C OK31.4 U1.58
GBM31: LED32.C OK32.4 U1.59
GLC1N: JP19.1 JP20.1 JP21.1 JP22.1 JP23.1 JP24.1 JP25.1 JP26.1 JP27.1 JP28.1 JP29.1 JP30.1 JP31.1 JP32.1 JP33.1 JP34.1 JP35.1
GLC1P: D65.A D67.C D69.A D71.C D73.A D75.C D77.A D79.C D81.A D83.C D85.A D87.C D89.A D91.C D93.A D95.C D97.A D99.C D101.A D103.C D105.A D107.C D109.A D111.C D113.A D115.C D117.A D119.C D121.A D123.C D125.A D127.C JP21.2 R19.1 R20.1 R21.1 R22.1 R23.1 R24.1 R25.1 R26.1 R27.1 R28.1 R29.1 R30.1 R31.1 R32.1 R33.1 R34.1
GLCN: JP1.1 JP2.1 JP4.1 JP5.1 JP6.1 JP7.1 JP8.1 JP9.1 JP10.1 JP11.1 JP12.1 JP13.1 JP14.1 JP15.1 JP16.1 JP17.1 JP18.1
GLCP: D1.A D3.C D5.A D7.C D9.A D11.C D13.A D15.C D17.A D19.C D21.A D23.C D25.A D27.C D29.A D31.C D33.A D35.C D37.A D39.C D41.A D43.C D45.A D47.C D49.A D51.C D53.A D55.C D57.A D59.C D61.A D63.C JP4.2 R1.1 R2.1 R5.1 R6.1 R7.1 R8.1 R9.1 R10.1 R11.1 R12.1 R13.1 R14.1 R15.1 R16.1 R17.1 R18.1
GND: C1.- C2.- C3.2 C4.2 C5.2 C6.2 C9.2 C10.2 IC1.1 JP3.5 JP36.3 OK1.3 OK2.3 OK3.3 OK4.3 OK5.3 OK6.3 OK7.3 OK8.3 OK9.3 OK10.3 OK11.3 OK12.3 OK13.3 OK14.3 OK15.3 OK16.3 OK17.3 OK18.3 OK19.3 OK20.3 OK21.3 OK22.3 OK23.3 OK24.3 OK25.3 OK26.3 OK27.3 OK28.3 OK29.3 OK30.3 OK31.3 OK32.3 S1.3 S1.4 SJ1.1 SJ4.1 U1.12 U1.18 U1.31 U1.47 U1.63 X1.3 X1.5 X2.3 X2.5
GND1 [Power]: C7.2 C8.2 C11.- C12.- C13.- C14.2 C15.2 C16.2 IC2.5 IC3.GND IC4.5 J1.2 JP37.1 JP38.3 JP39.1 R74.1 R75.1
GND2 [Power]: C17.2 C18.2 C19.- C20.- C21.- C22.2 C23.2 C24.2 IC5.5 IC6.GND IC7.5 J2.2 JP40.1 JP41.3 JP42.1 R84.1 R85.1
I2C_SCL: JP3.1 R67.1 U1.61
I2C_SDA: JP3.2 R68.1 U1.62
MES: C8.1 IC2.18 R77.2
MES1: C18.1 IC5.18 R87.2
N$1: R65.1 SJ1.2 U1.60
N$2: D3.A D4.C
N$3: D1.C D2.A
N$4: D2.C D4.A JP1.2 OK1.2
N$5: OK1.1 R1.2
N$6: D19.A D20.C
N$7: D7.A D8.C
N$8: D5.C D6.A
N$9: D6.C D8.A JP2.2 OK2.2
N$10: OK2.1 R2.2
N$11: D11.A D12.C
N$12: LED17.A R49.1
N$13: IC4.6 J1.4
N$14: LED1.A R3.1
N$15: C10.1 R66.1 S1.1 S1.2 U1.7
N$16: LED2.A R4.1
N$17: D9.C D10.A
N$18: D10.C D12.A JP5.2 OK3.2
N$19: OK3.1 R5.2
N$20: D17.C D18.A
N$21: D15.A D16.C
N$22: D13.C D14.A
N$23: D14.C D16.A JP6.2 OK4.2
N$24: OK4.1 R6.2
N$25: D18.C D20.A JP7.2 OK5.2
N$26: OK5.1 R7.2
N$27: D23.A D24.C
N$28: D21.C D22.A
N$29: D22.C D24.A JP8.2 OK6.2
N$30: OK6.1 R8.2
N$31: D27.A D28.C
N$32: D25.C D26.A
N$33: D26.C D28.A JP9.2 OK7.2
N$34: OK7.1 R9.2
N$35: D31.A D32.C
N$36: D29.C D30.A
N$37: D30.C D32.A JP10.2 OK8.2
N$38: OK8.1 R10.2
N$39: D35.A D36.C
N$40: D33.C D34.A
N$41: D34.C D36.A JP11.2 OK9.2
N$42: OK9.1 R11.2
N$43: D39.A D40.C
N$44: D37.C D38.A
N$45: D38.C D40.A JP12.2 OK10.2
N$46: OK10.1 R12.2
N$47: D43.A D44.C
N$48: D41.C D42.A
N$49: D42.C D44.A JP13.2 OK11.2
N$50: OK11.1 R13.2
N$51: D47.A D48.C
N$52: D45.C D46.A
N$53: D46.C D48.A JP14.2 OK12.2
N$54: OK12.1 R14.2
N$55: D51.A D52.C
N$56: D49.C D50.A
N$57: D50.C D52.A JP15.2 OK13.2
N$58: OK13.1 R15.2
N$59: D55.A D56.C
N$60: D53.C D54.A
N$61: D54.C D56.A JP16.2 OK14.2
N$62: OK14.1 R16.2
N$63: D59.A D60.C
N$64: D57.C D58.A
N$65: D58.C D60.A JP17.2 OK15.2
N$66: OK15.1 R17.2
N$67: D63.A D64.C
N$68: D61.C D62.A
N$69: D62.C D64.A JP18.2 OK16.2
N$70: OK16.1 R18.2
N$71: D67.A D68.C
N$72: D65.C D66.A
N$73: D66.C D68.A JP19.2 OK17.2
N$74: OK17.1 R19.2
N$75: D71.A D72.C
N$76: D69.C D70.A
N$77: D70.C D72.A JP20.2 OK18.2
N$78: OK18.1 R20.2
N$79: D75.A D76.C
N$80: D73.C D74.A
N$81: D74.C D76.A JP22.2 OK19.2
N$82: OK19.1 R21.2
N$83: D79.A D80.C
N$84: D77.C D78.A
N$85: D78.C D80.A JP23.2 OK20.2
N$86: OK20.1 R22.2
N$87: IC4.7 J1.3
N$88: D83.A D84.C
N$89: D81.C D82.A
N$90: D82.C D84.A JP24.2 OK21.2
N$91: OK21.1 R23.2
N$92: D87.A D88.C
N$93: D85.C D86.A
N$94: D86.C D88.A JP25.2 OK22.2
N$95: OK22.1 R24.2
N$96: D91.A D92.C
N$97: D89.C D90.A
N$98: D90.C D92.A JP26.2 OK23.2
N$99: OK23.1 R25.2
N$100: D95.A D96.C
N$101: D93.C D94.A
N$102: D94.C D96.A JP27.2 OK24.2
N$103: OK24.1 R26.2
N$104: D99.A D100.C
N$105: D97.C D98.A
N$106: D98.C D100.A JP28.2 OK25.2
N$107: OK25.1 R27.2
N$108: D103.A D104.C
N$109: D101.C D102.A
N$110: D102.C D104.A JP29.2 OK26.2
N$111: OK26.1 R28.2
N$112: D107.A D108.C
N$113: D105.C D106.A
N$114: D106.C D108.A JP30.2 OK27.2
N$115: OK27.1 R29.2
N$116: D111.A D112.C
N$117: D109.C D110.A
N$118: D110.C D112.A JP31.2 OK28.2
N$119: OK28.1 R30.2
N$120: D115.A D116.C
N$121: D113.C D114.A
N$122: D114.C D116.A JP32.2 OK29.2
N$123: OK29.1 R31.2
N$124: D119.A D120.C
N$125: D117.C D118.A
N$126: D118.C D120.A JP33.2 OK30.2
N$127: OK30.1 R32.2
N$128: D123.A D124.C
N$129: D121.C D122.A
N$130: D122.C D124.A JP34.2 OK31.2
N$131: OK31.1 R33.2
N$132: D127.A D128.C
N$133: D125.C D126.A
N$134: D126.C D128.A JP35.2 OK32.2
N$135: OK32.1 R34.2
N$136: IC7.6 J2.4
N$137: LED3.A R35.1
N$138: IC7.7 J2.3
N$139: LED4.A R36.1
N$141: LED5.A R37.1
N$143: LED6.A R38.1
N$145: LED7.A R39.1
N$147: LED8.A R40.1
N$149: LED9.A R41.1
N$151: LED10.A R42.1
N$153: LED11.A R43.1
N$155: LED12.A R44.1
N$157: LED13.A R45.1
N$159: LED14.A R46.1
N$161: LED15.A R47.1
N$163: LED16.A R48.1
N$164: LED18.A R50.1
N$165: LED19.A R51.1
N$166: LED20.A R52.1
N$167: LED21.A R53.1
N$168: LED22.A R54.1
N$169: LED23.A R55.1
N$170: LED24.A R56.1
N$171: LED25.A R57.1
N$172: LED26.A R58.1
N$173: LED27.A R59.1
N$174: LED28.A R60.1
N$175: LED29.A R61.1
N$176: LED30.A R62.1
N$177: LED31.A R63.1
N$178: LED32.A R64.1
POT: C13.+ IC2.1 JP38.2
POT1: C21.+ IC5.1 JP41.2
POTH: JP38.1 R78.2
POTH1: JP41.1 R88.2
PWM: IC2.9 R76.1
PWM1: IC5.9 R86.1
ROW1: D129.1 S2.1 S2.2 S3.1 S3.2 S4.1 S4.2 S5.1 S5.2
ROW2: D130.1 S6.1 S6.2 S7.1 S7.2 S8.1 S8.2 S9.1 S9.2
ROW3: D131.1 S10.1 S10.2 S11.1 S11.2 S12.1 S12.2 S13.1 S13.2
ROW4: D132.1 S14.1 S14.2 S15.1 S15.2 S16.1 S16.2 S17.1 S17.2
ROW5: D134.1 S18.1 S18.2 S19.1 S19.2 S20.1 S20.2 S21.1 S21.2
ROW6: D135.1 S22.1 S22.2 S23.1 S23.2 S24.1 S24.2 S25.1 S25.2
ROW7: D136.1 S26.1 S26.2 S27.1 S27.2 S28.1 S28.2 S29.1 S29.2
ROW8: D137.1 S30.1 S30.2 S31.1 S31.2 S32.1 S32.2 S33.1 S33.2
RS: IC2.16 JP37.4 JP39.4
RS1: IC5.16 JP40.4 JP42.4
RS232_RX: JP3.4 U1.30
RS232_TX: JP3.3 U1.29
RWN: JP37.5 JP39.5 R75.2
RWN1: JP40.5 JP42.5 R85.2
RX: IC2.7 IC4.1
RX1: IC5.7 IC7.1
S88N_CLK: U1.43 X1.4 X2.4
S88N_PS: U1.44 X1.6 X2.6
S88N_RAILDATA: U1.50 X1.8 X2.8
S88N_RST: U1.45 X1.7 X2.7
S88N_RX: U1.42 X1.2
S88N_TX: U1.41 X2.2
S88N_VCC: SJ3.2 X1.1 X2.1
SPI_CLK: JP3.7 U1.34
SPI_CS: JP3.8 U1.33
SPI_MISO: JP3.10 U1.35
SPI_MOSI: JP3.9 U1.36
SWCLK: JP36.2 U1.49
SWDIO: JP36.4 U1.46
TP: C7.1 R76.2 R77.1
TP1: C17.1 R86.2 R87.1
TX: IC2.8 IC4.4
TX1: IC5.8 IC7.4
V3_3: C2.+ C4.1 C5.1 C6.1 C9.1 IC1.2 JP3.6 JP36.1 R3.2 R4.2 R35.2 R36.2 R37.2 R38.2 R39.2 R40.2 R41.2 R42.2 R43.2 R44.2 R45.2 R46.2 R47.2 R48.2 R49.2 R50.2 R51.2 R52.2 R53.2 R54.2 R55.2 R56.2 R57.2 R58.2 R59.2 R60.2 R61.2 R62.2 R63.2 R64.2 R65.2 R66.2 R67.2 R68.2 SJ3.1 SJ4.2 U1.1 U1.13 U1.19 U1.32 U1.48 U1.64
V5_0: C1.+ C3.1 IC1.3 SJ3.3
VDD [Power]: C12.+ C15.1 C16.1 IC2.14 IC3.OUT IC4.8 JP37.2 JP39.2 R69.2 R70.2 R71.2 R72.2 R73.2 R78.1
VDD1 [Power]: C20.+ C23.1 C24.1 IC5.14 IC6.OUT IC7.8 JP40.2 JP42.2 R79.2 R80.2 R81.2 R82.2 R83.2 R88.1
VIN [Power]: C11.+ C14.1 D133.C IC3.IN
VIN1 [Power]: C19.+ C22.1 D138.C IC6.IN
VO: JP37.3 JP39.3 R73.1 R74.2
VO1: JP40.3 JP42.3 R83.1 R84.2
XVDD [Power]: D133.A J1.5
XVDD1 [Power]: D138.A J2.5

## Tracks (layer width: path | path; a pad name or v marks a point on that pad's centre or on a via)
COL1
  Top 0.254: S14.3 101.52,96.6 101.52,90.2 S14.4 | S10.3 109.12,96.6 109.12,90.2 S10.4 | S6.3 116.72,96.6 116.72,90.2 S6.4 | S2.3 124.32,96.6 124.32,90.2 S2.4
  Bottom 0.254: IC2.17 141.02,86.6 139.12,84.7 135.02,84.7 134.12,85.6 131.12,85.6 128.52,88.2 127.22,88.2 126.92,88.5 R69.1 126.82,88.6 125.32,90.1 124.42,90.1 S2.4 124.32,90.1 122.42,88.2 118.72,88.2 118.67,88.25 | 118.67,88.25 116.82,90.1 S6.4 | 110.97,88.25 111.02,88.2 118.62,88.2 118.67,88.25 | 110.97,88.25 109.12,90.1 S10.4 | S14.4 101.52,90.1 103.42,88.2 110.92,88.2 110.97,88.25
COL2
  Top 0.254: S15.3 101.52,85.4 101.52,79 S15.4 | S11.3 109.12,85.4 109.12,79 S11.4 | S7.3 116.72,85.4 116.72,79 S7.4 | S3.4 124.32,79 124.32,85.4 S3.3
  Bottom 0.254: 125.92,83 125.92,83.1 125.37,83.65 | 125.92,83 125.92,82.4 R70.1 | 125.37,83.65 124.42,84.6 124.42,85.4 S3.3 | 125.92,83 126.62,83 127.02,83.4 129.12,83.4 129.52,83.8 133.12,83.8 133.42,84.1 IC2.3 | 118.57,83.65 118.62,83.6 125.32,83.6 125.37,83.65 | 118.57,83.65 116.82,85.4 S7.3 | 110.87,83.65 110.92,83.6 118.52,83.6 118.57,83.65 | 110.87,83.65 109.12,85.4 S11.3 | S15.3 101.52,85.4 103.32,83.6 110.82,83.6 110.87,83.65
COL3
  Top 0.254: S16.3 101.52,74.3 101.52,67.9 S16.4 | S12.4 109.12,67.9 109.12,74.3 S12.3 | S4.3 124.32,74.3 124.32,67.9 S4.4 | IC2.4 133.42,81.6 127.22,81.6 127.22,96.1 124.82,98.5 117.92,98.5 117.92,75.5 116.82,74.4 S8.3 116.72,74.2 116.72,67.9 S8.4
  Bottom 0.254: R71.1 125.92,71 125.02,71.9 111.52,71.9 109.12,74.3 S12.3 | S16.4 101.52,67.8 103.42,65.9 107.12,65.9 109.02,67.8 S12.4 109.22,67.8 111.12,65.9 118.72,65.9 | 118.72,65.9 122.42,65.9 124.32,67.8 S4.4 | 118.72,65.9 116.82,67.8 S8.4
COL4  (via drill 0.61)
  Top 0.254: S13.3 109.12,63.1 109.12,56.7 S13.4 | S17.3 101.52,63.1 101.52,56.7 S17.4 | S5.4 124.32,56.7 124.32,63.1 S5.3 | v119.22,77.5 118.42,76.7 118.42,64.8 116.82,63.2 S9.3 116.72,63.1 116.72,56.7 S9.4
  Bottom 0.254: S17.3 101.52,63.1 103.42,61.2 107.12,61.2 109.02,63.1 S13.3 109.22,63.1 111.12,61.2 118.72,61.2 | R72.1 125.92,60 125.92,63.1 124.42,63.1 S5.3 124.32,63.1 122.42,61.2 118.72,61.2 | v119.22,77.5 119.62,77.1 132.82,77.1 133.42,76.5 IC2.6 | 118.72,61.2 116.82,63.1 S9.3
COL5
  Top 0.254: S30.3 101.52,44.6 101.52,38.2 S30.4 | S26.3 109.12,44.6 109.12,38.2 S26.4 | S22.3 116.72,44.6 116.72,38.2 S22.4 | S18.3 124.32,44.6 124.32,38.2 S18.4
  Bottom 0.254: IC5.17 141.02,34.6 139.12,32.7 135.02,32.7 134.12,33.6 131.12,33.6 128.52,36.2 127.22,36.2 126.92,36.5 R79.1 126.82,36.6 125.32,38.1 124.42,38.1 S18.4 124.32,38.1 122.42,36.2 118.72,36.2 118.67,36.25 | 118.67,36.25 116.82,38.1 S22.4 | 110.97,36.25 111.02,36.2 118.62,36.2 118.67,36.25 | 110.97,36.25 109.12,38.1 S26.4 | S30.4 101.52,38.1 103.42,36.2 110.92,36.2 110.97,36.25
COL6
  Top 0.254: S31.3 101.52,33.4 101.52,27 S31.4 | S27.3 109.12,33.4 109.12,27 S27.4 | S23.3 116.72,33.4 116.72,27 S23.4 | S19.4 124.32,27 124.32,33.4 S19.3
  Bottom 0.254: 125.92,31 125.92,31.1 125.37,31.65 | 125.92,31 125.92,30.4 R80.1 | 125.37,31.65 124.42,32.6 124.42,33.4 S19.3 | 125.92,31 126.62,31 127.02,31.4 129.12,31.4 129.52,31.8 133.12,31.8 133.42,32.1 IC5.3 | 118.57,31.65 118.62,31.6 125.32,31.6 125.37,31.65 | 118.57,31.65 116.82,33.4 S23.3 | 110.87,31.65 110.92,31.6 118.52,31.6 118.57,31.65 | 110.87,31.65 109.12,33.4 S27.3 | S31.3 101.52,33.4 103.32,31.6 110.82,31.6 110.87,31.65
COL7
  Top 0.254: S32.3 101.52,22.3 101.52,15.9 S32.4 | S28.4 109.12,15.9 109.12,22.3 S28.3 | S20.3 124.32,22.3 124.32,15.9 S20.4 | IC5.4 133.42,29.6 127.22,29.6 127.22,44.1 124.82,46.5 117.92,46.5 117.92,23.5 116.82,22.4 S24.3 116.72,22.2 116.72,15.9 S24.4
  Bottom 0.254: R81.1 125.92,19 125.02,19.9 111.52,19.9 109.12,22.3 S28.3 | S32.4 101.52,15.8 103.42,13.9 107.12,13.9 109.02,15.8 S28.4 109.22,15.8 111.12,13.9 118.72,13.9 | 118.72,13.9 122.42,13.9 124.32,15.8 S20.4 | 118.72,13.9 116.82,15.8 S24.4
COL8  (via drill 0.61)
  Top 0.254: S29.3 109.12,11.1 109.12,4.7 S29.4 | S33.3 101.52,11.1 101.52,4.7 S33.4 | S21.4 124.32,4.7 124.32,11.1 S21.3 | v119.22,25.5 118.42,24.7 118.42,12.8 116.82,11.2 S25.3 116.72,11.1 116.72,4.7 S25.4
  Bottom 0.254: S33.3 101.52,11.1 103.42,9.2 107.12,9.2 109.02,11.1 S29.3 109.22,11.1 111.12,9.2 118.72,9.2 | R82.1 125.92,8 125.92,11.1 124.42,11.1 S21.3 124.32,11.1 122.42,9.2 118.72,9.2 | v119.22,25.5 119.62,25.1 132.82,25.1 133.42,24.5 IC5.6 | 118.72,9.2 116.82,11.1 S25.3
DB1  (via drill 0.61)
  Top 0.254: v102.72,42.7 104.82,40.6 104.82,3.5 106.12,2.2 144.22,2.2 144.22,9.8 | 144.22,9.8 144.22,11 143.42,11.8 142.92,11.8 141.12,13.6 141.12,16.8 IC5.10 | JP40.11 146.12,32.4 147.42,31.1 147.42,27.5 149.02,25.9 149.02,16.2 148.22,15.4 148.22,14.2 146.92,12.9 146.92,12.4 144.32,9.8 144.22,9.8
  Bottom 0.254: JP42.11 156.82,32.6 155.52,31.3 147.82,31.3 146.72,32.4 146.12,32.4 JP40.11 | v102.72,42.7 103.82,42.7 103.92,42.8 D137.3
DB2  (via drill 0.61)
  Top 0.254: v152.42,33.4 149.72,30.7 v149.72,27.6 | v118.92,37.2 120.12,36 v120.12,13 | JP40.13 146.12,29.8 146.52,29.4 146.52,24.9 145.52,23.9 145.52,21.7 146.12,21.1 146.12,15.3 145.12,14.3 142.82,14.3 142.82,20.2 141.12,21.9 IC5.12
  Bottom 0.254: v152.42,33.4 152.52,33.4 156.82,37.7 JP42.13 | v149.72,27.6 145.02,27.6 144.42,28.2 144.42,29.1 144.72,29.1 145.42,29.8 146.02,29.8 JP40.13 | v118.92,37.2 118.92,42.6 D135.3 | v120.12,13 120.52,13.4 135.52,13.4 140.52,18.4 142.22,18.4 142.82,19 142.82,21.9 141.12,21.9 IC5.12
DB3  (via drill 0.61)
  Top 0.254: v114.52,42.2 115.22,41.5 v115.22,21.5 | v139.02,29.6 138.72,29.3 138.72,21.8 141.02,19.5 IC5.11
  Bottom 0.254: JP42.12 156.82,35.1 154.22,32.5 148.62,32.5 JP40.12 148.52,32.5 147.42,33.6 144.72,33.6 141.72,30.6 140.02,30.6 v139.02,29.6 | v114.52,42.2 111.62,42.2 111.42,42.4 D136.3 | v115.22,21.5 116.32,20.4 126.02,20.4 126.82,21.2 127.62,21.2 128.42,20.4 132.32,20.4 132.42,20.5 140.02,20.5 141.02,19.5 IC5.11
DB4  (via drill 0.61)
  Top 0.254: v102.72,94.7 104.82,92.6 104.82,55.5 106.12,54.2 144.22,54.2 144.22,61.8 | 144.22,61.8 144.22,63 143.42,63.8 142.92,63.8 141.12,65.6 141.12,68.8 IC2.10 | JP37.11 146.12,84.4 147.42,83.1 147.42,79.5 149.02,77.9 149.02,68.2 148.22,67.4 148.22,66.2 146.92,64.9 146.92,64.4 144.32,61.8 144.22,61.8
  Bottom 0.254: JP39.11 156.82,84.6 155.52,83.3 147.82,83.3 146.72,84.4 146.12,84.4 JP37.11 | v102.72,94.7 103.82,94.7 103.92,94.8 D132.3
DB5  (via drill 0.61)
  Top 0.254: v114.52,94.2 115.22,93.5 v115.22,73.5 | v139.02,81.6 138.72,81.3 138.72,73.8 141.02,71.5 IC2.11
  Bottom 0.254: JP39.12 156.82,87.1 154.22,84.5 148.62,84.5 JP37.12 148.52,84.5 147.42,85.6 144.72,85.6 141.72,82.6 140.02,82.6 v139.02,81.6 | v114.52,94.2 111.62,94.2 111.42,94.4 D131.3 | v115.22,73.5 116.32,72.4 126.02,72.4 126.82,73.2 127.62,73.2 128.42,72.4 132.32,72.4 132.42,72.5 140.02,72.5 141.02,71.5 IC2.11
DB6  (via drill 0.61)
  Top 0.254: v152.42,85.4 149.72,82.7 v149.72,79.6 | v118.92,89.2 120.12,88 v120.12,65 | JP37.13 146.12,81.8 146.52,81.4 146.52,76.9 145.52,75.9 145.52,73.7 146.12,73.1 146.12,67.3 145.12,66.3 142.82,66.3 142.82,72.2 141.12,73.9 IC2.12
  Bottom 0.254: v152.42,85.4 152.52,85.4 156.82,89.7 JP39.13 | v149.72,79.6 145.02,79.6 144.42,80.2 144.42,81.1 144.72,81.1 145.42,81.8 146.02,81.8 JP37.13 | v118.92,89.2 118.92,94.6 D130.3 | v120.12,65 120.52,65.4 135.52,65.4 140.52,70.4 142.22,70.4 142.82,71 142.82,73.9 141.12,73.9 IC2.12
DB7  (via drill 0.61)
  Top 0.254: v139.62,80.3 139.32,80 139.32,78.2 141.02,76.5 IC2.13 | JP39.14 156.82,92.3 151.92,97.2 151.92,98.8 146.12,98.8 v138.12,90.8 138.12,83.1 v137.22,82.2
  Bottom 0.254: JP37.14 148.52,81.9 147.42,83 145.62,83 143.12,80.5 139.82,80.5 v139.62,80.3 139.52,80.3 139.12,80.7 138.72,80.7 v137.22,82.2 | v138.12,90.8 132.92,90.8 129.42,94.3 126.92,94.3 126.42,94.8 D129.3
DB8  (via drill 0.61)
  Top 0.254: v139.62,28.3 139.32,28 139.32,26.2 141.02,24.5 IC5.13 | JP42.14 156.82,40.3 151.92,45.2 151.92,46.8 146.12,46.8 v138.12,38.8 138.12,31.1 v137.22,30.2
  Bottom 0.254: JP40.14 148.52,29.9 147.42,31 145.62,31 143.12,28.5 139.82,28.5 v139.62,28.3 139.52,28.3 139.12,28.7 138.72,28.7 v137.22,30.2 | v138.12,38.8 132.92,38.8 129.42,42.3 126.92,42.3 126.42,42.8 D134.3
DIR  (via drill 0.61)
  Top 0.254: v130.32,98 130.32,90.2 132.62,87.9 132.62,87.5 133.42,86.7 IC2.2 | v110.62,96 110.22,95.6 110.22,88.9 107.52,86.2 v107.52,73.5
  Bottom 0.254: v130.32,98 129.82,98.5 113.12,98.5 v110.62,96 | v107.52,73.5 106.42,72.4 100.12,72.4 99.42,73.1 91.82,73.1 90.82,72.1 IC4.2 90.82,71.9 90.82,69.5 IC4.3
DIR1  (via drill 0.61)
  Top 0.254: v130.32,46 130.32,38.2 132.62,35.9 132.62,35.5 133.42,34.7 IC5.2 | v110.62,44 110.22,43.6 110.22,36.9 107.52,34.2 v107.52,21.5
  Bottom 0.254: v130.32,46 129.82,46.5 113.12,46.5 v110.62,44 | v107.52,21.5 106.42,20.4 100.12,20.4 99.42,21.1 91.82,21.1 90.82,20.1 IC7.2 90.82,19.9 90.82,17.5 IC7.3
E  (via drill 0.61)
  Top 0.254: 139.42,83.2 141.02,81.6 IC2.15 | v139.42,87.6 139.42,83.2 | v154.02,71.9 152.42,70.3 v152.42,65.4 | v143.32,62.7 138.12,67.9 138.12,82 139.32,83.2 139.42,83.2
  Bottom 0.254: v139.42,87.6 139.92,88.1 143.12,88.1 145.92,90.9 146.72,90.9 147.82,92 148.52,92 JP37.6 | v154.02,71.9 156.82,71.9 JP39.6 | v152.42,65.4 149.72,62.7 v143.32,62.7
E1  (via drill 0.61)
  Top 0.254: 139.42,31.2 141.02,29.6 IC5.15 | v139.42,35.6 139.42,31.2 | v154.02,19.9 152.42,18.3 v152.42,13.4 | v143.32,10.7 138.12,15.9 138.12,30 139.32,31.2 139.42,31.2
  Bottom 0.254: v139.42,35.6 139.92,36.1 143.12,36.1 145.92,38.9 146.72,38.9 147.82,40 148.52,40 JP40.6 | v154.02,19.9 156.82,19.9 JP42.6 | v152.42,13.4 149.72,10.7 v143.32,10.7
GBM0  (via drill 0.5)
  Top 0.2: LED1.C 5.81,65.7 5.11,65.7 OK1.4 | v8.31,59 19.61,59 20.61,58 21.21,58 21.71,58.5 25.61,58.5 25.91,58.2 36.58,58.2 37.21,57.56 37.21,56.3 U1.14
  Bottom 0.2: v8.31,59 5.11,62.2 5.11,65.7 OK1.4
GBM1  (via drill 0.5)
  Top 0.2: LED2.C 6.81,65.7 7.61,65.7 OK2.4 | v30.21,59.4 30.01,59.6 15.91,59.6 15.71,59.4 9.11,59.4 v8.31,60.2 | U1.15 36.71,56.2 36.71,57.1 36.51,57.3 31.51,57.3 v31.41,57.4
  Bottom 0.2: v31.41,57.4 30.21,58.6 v30.21,59.4 | v8.31,60.2 7.71,60.8 7.71,65.7 OK2.4
GBM2  (via drill 0.5)
  Top 0.2: LED3.C 16.01,65.7 15.31,65.7 OK3.4 | v31.31,59.4 30.51,60.2 v15.41,60.2 | U1.16 32.94,56.23 v32.51,56.4
  Bottom 0.2: v31.31,59.4 31.31,58.8 32.51,57.5 v32.51,56.4 | v15.41,60.2 15.31,60.3 15.31,65.7 OK3.4
GBM3  (via drill 0.5)
  Top 0.2: LED4.C 17.01,65.7 17.71,65.7 OK4.4 | U1.17 34.21,54.3 33.61,54.9 28.61,54.9 27.61,55.9 19.21,55.9 v18.91,56.2
  Bottom 0.2: v18.91,56.2 17.81,57.3 17.81,65.7 OK4.4
GBM4  (via drill 0.5)
  Top 0.2: LED5.C 26.21,65.7 OK5.4 | v32.31,52.8 34.21,52.8 U1.20
  Bottom 0.2: v32.31,52.8 29.41,55.7 29.41,61.5 25.41,65.5 OK5.4
GBM5  (via drill 0.5)
  Top 0.2: LED6.C 27.21,65.7 27.91,65.7 OK6.4 | v35.51,52.1 35.31,52.3 34.31,52.3 U1.21
  Bottom 0.2: v35.51,52.1 34.11,53.5 34.11,59.7 30.31,63.5 28.01,63.5 28.01,65.7 OK6.4
GBM6  (via drill 0.5)
  Top 0.2: LED7.C 36.31,65.7 35.61,65.7 OK7.4 | v32.91,51.8 34.21,51.8 U1.22 | v33.31,59.4 34.71,59.4 v35.51,60.2
  Bottom 0.2: v32.91,51.8 33.31,52.2 v33.31,59.4 | v35.51,60.2 35.51,65.7 OK7.4
GBM7  (via drill 0.5)
  Top 0.2: LED8.C 37.31,65.7 OK8.4 | v38.51,51.1 38.31,51.3 34.31,51.3 U1.23
  Bottom 0.2: v38.51,51.1 40.21,52.8 40.21,53.8 41.01,54.6 41.01,62.2 38.11,65.1 OK8.4
GBM8  (via drill 0.5)
  Top 0.2: LED9.C 46.51,65.7 45.81,65.7 OK9.4 | v42.61,60.3 43.51,61.2 v45.41,61.2 | U1.39 39.19,45.92 v38.91,46.2
  Bottom 0.2: v45.41,61.2 45.71,61.5 45.71,65.7 OK9.4 | v38.91,46.2 38.91,48 42.21,51.3 42.21,59.9 v42.61,60.3
GBM9  (via drill 0.5)
  Top 0.2: LED10.C 47.51,65.7 48.21,65.7 OK10.4 | U1.40 39.69,46.18 v40.11,46.6
  Bottom 0.2: OK10.4 48.21,65.8 48.21,67.8 44.31,67.8 43.81,67.3 43.81,66.7 44.11,66.4 44.11,64.1 43.41,63.4 43.51,63.3 43.51,55 42.81,54.3 42.81,50.8 40.11,48.1 v40.11,46.6
GBM10  (via drill 0.5)
  Top 0.2: 56.61,65.7 LED11.C | 56.61,65.7 55.91,65.7 OK11.4 | v66.21,50.8 65.41,50.8 64.71,51.5 51.11,51.5 51.11,49.9 49.01,47.8 45.71,47.8 U1.51 | v67.31,66.3 66.91,66.7 57.61,66.7 56.61,65.7
  Bottom 0.2: v66.21,50.8 67.31,51.9 v67.31,66.3
GBM11  (via drill 0.5)
  Top 0.2: LED12.C 57.71,65.7 58.41,65.7 OK12.4 | v57.31,54.4 54.81,51.9 50.71,51.9 50.71,50.1 48.91,48.3 45.71,48.3 U1.52
  Bottom 0.2: v57.31,54.4 59.31,56.4 59.31,64.9 58.51,65.7 OK12.4
GBM12  (via drill 0.5)
  Top 0.2: LED13.C 66.81,65.7 66.11,65.7 OK13.4 | v49.71,50.2 48.31,48.8 45.71,48.8 U1.53 | v57.51,75.4 58.01,75.9 71.11,75.9 72.11,74.9 72.11,70.4 v70.01,70.4
  Bottom 0.2: v49.71,50.2 51.61,52.1 51.61,63.4 52.41,64.2 52.41,68.5 57.51,73.6 v57.51,75.4 | v70.01,70.4 66.11,66.5 66.11,65.8 OK13.4
GBM13  (via drill 0.5)
  Top 0.2: LED14.C 67.81,65.7 68.11,65.7 | 68.11,65.7 68.51,65.7 OK14.4 68.11,65.7 | v44.31,57.3 43.21,57.3 43.21,56.3 U1.2 | v44.61,67 44.71,67.1 67.61,67.1 68.11,66.6 68.11,65.7
  Bottom 0.2: v44.31,57.3 44.61,57.6 v44.61,67
GBM14  (via drill 0.5)
  Top 0.2: LED15.C 77.01,65.7 OK15.4 | v53.61,55.7 52.71,54.8 52.11,54.8 51.81,55.1 47.11,55.1 46.61,55.6 46.61,56.3 44.81,58.1 43.41,58.1 42.71,57.4 42.71,56.2 U1.3 | v61.11,69.7 63.81,72.4 63.91,72.4 65.11,73.6 65.11,75.5 69.01,75.5 70.21,74.3 70.21,71.9 v70.71,71.9
  Bottom 0.2: v53.61,55.7 55.21,57.3 55.21,60.5 57.51,62.8 57.51,66.1 v61.11,69.7 | v70.71,71.9 76.21,66.4 OK15.4
GBM15
  Top 0.2: LED16.C 50.91,58.9 50.51,59.3 49.61,59.3 OK16.4 49.51,59.3 47.91,57.7 47.11,57.7 46.71,58.1 45.41,58.1 44.91,58.6 42.71,58.6 42.21,58.1 42.21,56.3 U1.4
GBM16  (via drill 0.5)
  Top 0.2: LED17.C 73.11,37.7 73.11,35.3 73.61,35.3 OK17.4 | v40.21,54.9 40.21,56.2 U1.8 | v38.01,33.3 38.21,33.5 v71.91,33.5
  Bottom 0.2: v40.21,54.9 39.31,54 39.31,53 36.71,50.4 36.71,34.2 36.11,33.6 36.11,33 36.61,32.5 38.01,32.5 v38.01,33.3 | v71.91,33.5 73.61,35.2 OK17.4
GBM17  (via drill 0.5)
  Top 0.2: LED18.C 71.81,37.7 71.81,35.3 71.21,35.3 OK18.4 | v52.41,61.2 48.81,61.2 47.11,59.5 40.35,59.5 39.71,58.87 39.71,56.3 U1.9 | v54.91,68.3 55.21,68.6 60.31,68.6 60.41,68.7 65.31,68.7 66.51,67.5 v70.71,67.5
  Bottom 0.2: v52.41,61.2 54.91,63.7 v54.91,68.3 | v70.71,67.5 72.51,65.7 72.51,52.4 74.11,51.2 74.11,44.5 72.21,42.6 72.21,41.4 71.21,40.4 71.21,35.3 OK18.4
GBM18  (via drill 0.5)
  Top 0.2: LED19.C 62.71,37.7 62.71,35.3 63.51,35.3 OK19.4 | v20.91,58.8 21.01,58.9 25.81,58.9 26.11,58.6 38.96,58.6 39.21,58.35 39.21,56.3 U1.10 | v49.51,25.9 50.01,25.4 56.21,25.4 57.51,26.7 57.51,29.8 v58.11,29.8
  Bottom 0.2: v20.91,58.8 20.61,58.5 20.61,46.1 19.11,44.6 19.11,29.6 20.11,28.6 49.26,28.6 49.51,28.35 v49.51,25.9 | v58.11,29.8 63.51,35.2 OK19.4
GBM19  (via drill 0.5)
  Top 0.2: 61.51,35.3 61.51,37.7 LED20.C | 61.51,35.3 61.01,35.3 OK20.4 61.51,35.3 | v38.41,57.8 38.46,57.8 38.71,57.55 38.71,56.3 U1.11 | v64.41,34.3 62.51,34.3 61.51,35.3
  Bottom 0.2: v38.41,57.8 36.91,59.3 36.91,87.8 37.81,88.7 39.51,88.7 39.51,93 40.21,93.7 40.21,94 41.01,94.8 66.91,94.8 66.91,93.1 69.91,90.1 69.91,71.6 74.91,66.6 74.91,56.1 76.61,54.4 76.61,40.7 72.11,36.2 72.11,34.9 71.51,34.3 v64.41,34.3
GBM20  (via drill 0.5)
  Top 0.2: 52.61,35.3 52.61,37.7 LED21.C | 52.61,35.3 53.31,35.3 OK21.4 | v29.21,35.2 30.31,34.1 39.81,34.1 40.01,33.9 51.21,33.9 52.61,35.3 | U1.24 34.21,50.8 31.51,50.8 29.81,49.1 v26.91,49.1
  Bottom 0.2: v26.91,49.1 27.11,48.9 27.11,38.6 29.21,36.5 v29.21,35.2
GBM21  (via drill 0.5)
  Top 0.2: LED22.C 51.51,37.6 51.51,35.3 50.81,35.3 OK22.4 | v37.71,50.3 34.31,50.3 U1.25 | v49.61,41 49.21,41.4 43.61,41.4 43.21,41 42.61,41 41.71,41.9 41.31,41.9 41.01,41.6 v39.81,41.6
  Bottom 0.2: v49.61,41 50.81,39.8 OK22.4 | v39.81,41.6 39.81,42.6 40.31,43.1 40.31,43.9 39.71,44.4 38.11,44.4 38.11,48.5 38.31,48.7 38.31,49.7 v37.71,50.3
GBM22  (via drill 0.5)  (1 unrouted)
  Top 0.2: LED23.C 42.51,37.7 42.51,35.3 43.11,35.3 OK23.4 | v38.71,41.4 38.21,41.8 38.21,44.8 U1.37
  Bottom 0.2: v38.71,41.4 38.71,40.4 39.61,39.5 39.61,33.4 41.11,31.9 42.41,31.9 42.71,32.2 42.71,34.7 43.21,35.2
GBM23  (via drill 0.5)
  Top 0.2: LED24.C 41.41,37.7 41.41,35.3 40.71,35.3 OK24.4 | 38.71,44.8 U1.38 38.71,44.81 38.71,43 39.11,42.6 40.51,42.6 v40.71,42.4
  Bottom 0.2: 40.71,35.29 OK24.4 40.11,35.77 40.11,40.8 40.61,41.3 40.61,42.3 v40.71,42.4
GBM24  (via drill 0.5)
  Top 0.2: LED25.C 32.41,37.8 32.41,35.3 33.01,35.3 OK25.4 | U1.26 32.59,49.78 v32.31,49.5
  Bottom 0.2: OK25.4 33.11,35.3 33.91,36.1 33.91,44.6 31.91,46.6 31.91,49.1 v32.31,49.5
GBM25  (via drill 0.5)
  Top 0.2: LED26.C 31.21,37.8 31.21,35.3 30.51,35.3 OK26.4 | U1.27 34.21,49.3 33.51,49.3 32.91,48.7 v30.51,48.7
  Bottom 0.2: v30.51,48.7 30.51,35.3 OK26.4
GBM26  (via drill 0.5)
  Top 0.2: LED27.C 22.21,37.7 22.21,35.3 22.81,35.3 OK27.4 | v37.51,49.1 37.21,48.8 34.31,48.8 U1.28 | v36.91,33.3 36.71,33.5 v24.01,33.5
  Bottom 0.2: v37.51,49.1 37.11,48.7 37.11,33.5 v36.91,33.3 | v24.01,33.5 22.91,34.6 22.91,35.2 OK27.4
GBM27  (via drill 0.5)
  Top 0.2: LED28.C 21.11,37.7 21.11,35.3 20.41,35.3 OK28.4 | v48.51,50.1 47.91,49.5 46.61,49.5 46.31,49.8 45.71,49.8 U1.55
  Bottom 0.2: v48.51,50.1 48.11,49.7 48.11,37.6 47.11,36.6 47.11,32.2 43.91,29 20.61,29 19.61,30 19.61,34.5 20.31,35.2 OK28.4
GBM28  (via drill 0.5)
  Top 0.2: LED29.C 12.11,37.7 12.11,35.3 12.71,35.3 OK29.4 | v46.91,50.3 45.71,50.3 U1.56 | v46.91,88.3 46.81,88.4 v11.61,88.4
  Bottom 0.2: v46.91,50.3 46.71,50.5 46.71,55.5 46.61,55.6 46.61,61.5 49.21,64.1 49.21,71.1 46.91,73.4 v46.91,88.3 | v11.61,88.4 11.31,88.1 11.31,58.5 10.81,58 10.81,45 12.71,43.1 OK29.4
GBM29  (via drill 0.5)
  Top 0.2: LED30.C 10.91,37.7 10.91,35.3 10.21,35.3 OK30.4 | v36.31,52.9 37.11,52.1 40.01,52.1 41.31,50.8 45.61,50.8 U1.57
  Bottom 0.2: v36.31,52.9 34.51,54.7 34.51,59.9 31.41,63 31.41,68.5 26.61,73.3 26.61,87.8 25.71,88.7 24.21,88.7 24.21,92.9 24.51,93.2 24.51,94.1 23.81,94.8 13.11,94.8 13.11,93.3 12.41,92.6 10.11,92.6 10.11,91.3 8.71,89.9 8.71,89.4 7.81,88.5 6.41,88.5 6.41,68.3 9.11,65.6 9.11,36.3 10.11,35.3 OK30.4
GBM30  (via drill 0.5, 0.6)
  Top 0.2: LED31.C 2.01,37.7 2.01,35.3 2.51,35.3 OK31.4 | v37.41,52.9 37.81,52.5 40.21,52.5 41.41,51.3 45.61,51.3 U1.58 | v29.51,51.6 28.61,51.6 27.91,50.9 22.21,50.9 17.01,45.7 11.21,45.7 7.51,49.4 v7.51,49.7
  Bottom 0.2: v37.41,52.9 35.51,51 30.11,51 v29.51,51.6 | OK31.4 2.61,35.3 5.51,38.2 5.51,44.5 7.61,46.6 7.61,49.6 v7.51,49.7
GBM31  (via drill 0.5)
  Top 0.2: LED32.C 30.41,42.1 30.91,41.6 31.71,41.6 OK32.4 33.33,41.58 34.31,40.6 41.41,40.6 v41.71,40.8 | U1.59 44.03,51.78 v43.71,52.1
  Bottom 0.2: v43.71,52.1 43.71,49.2 41.61,47.1 41.61,46.2 42.41,45.4 42.41,43.6 41.91,43.1 41.91,41 v41.71,40.8
GLC1N
  Top 0.2: JP35.1 3.81,41.5 2.31,40 1.51,40 1.21,39.7 1.21,8.5 6.71,8.5 11.01,4.2 JP34.1
  Top 1.676: JP19.1 JP20.1 JP22.1 JP23.1 JP24.1 JP25.1 JP26.1 JP27.1 JP21.1 JP28.1 JP29.1 JP30.1 JP31.1 JP32.1 JP33.1 JP34.1
  pour Bottom: 71.01,5 71.01,0.5 0.51,0.5 0.51,46 19.01,46 19.01,5
GLC1P  (via drill 0.5)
